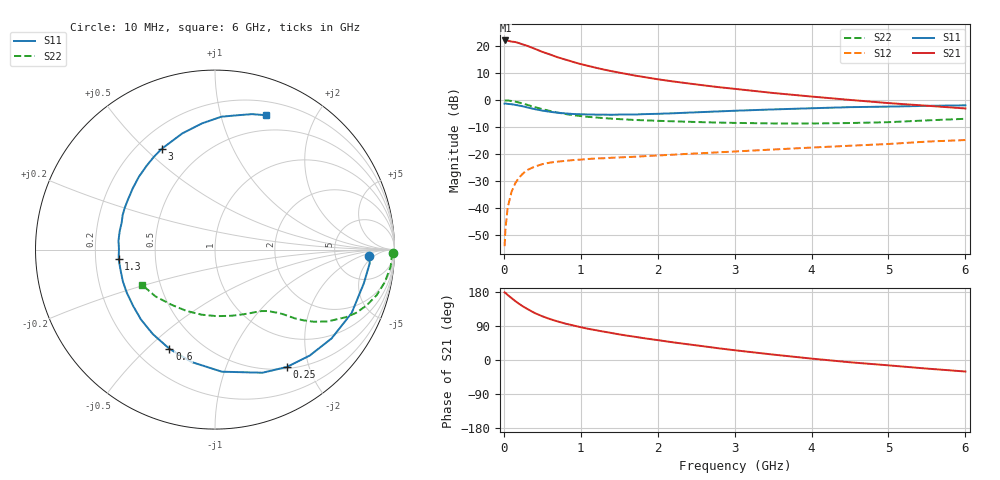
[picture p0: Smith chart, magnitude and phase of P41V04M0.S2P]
! SIEMENS Small Signal Semiconductors
! BFP182
! Si NPN RF Bipolar Junction Transistor in SOT143
! VCE = 1 V  IC = 4 mA
! Common Emitter S-Parameters:  March  1996
# GHz  S  MA  R  50
!  f  S11  S21  S12  S22
! GHz  MAG  ANG  MAG  ANG  MAG  ANG  MAG  ANG
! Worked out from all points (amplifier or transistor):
!   36 points, 10 MHz to 6 GHz, reference 50 ohm
!   highest |S21| = 22.0 dB at 20 MHz (marker M1)
!   |S21| within 3 dB of that: start of sweep to 395.9 MHz
!   unconditionally stable (mu >= 1): 1.622 GHz to end of sweep
!   at 250 MHz: K = 0.20, MSG = 23.8 dB, |S12| = -27.1 dB
!   at 1.4 GHz: K = 0.90, MSG = 16.0 dB, |S12| = -21.3 dB
!   at 6 GHz: K = 1.02, MAG = 4.9 dB, |S12| = -14.8 dB
!   S11 on the Smith chart (normalised r, x): 10 MHz: 12, -3; 250 MHz: 0.52, -1.66; 600 MHz: 0.34, -0.59; 1.3 GHz: 0.30, -0.04; 3 GHz: 0.30, +0.56; 6 GHz: 0.33, +1.40
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0.01  0.8606 -2.4  12.42 178.6  0.002 81.2  0.9895 -1.1
0.02  0.8652 -5.1  12.65 177.2  0.004 88.8  0.9859 -2.2
0.05  0.8504 -12.7  12.52 171.6  0.0104 84.8  0.9835 -5.5
0.15  0.8166 -37.3  11.81 155.3  0.0293 69.9  0.9356 -15.8
0.2  0.7919 -48.2  11.27 148.0  0.0374 65.0  0.9003 -20.2
0.25  0.7669 -58.5  10.62 141.2  0.0442 59.3  0.8621 -24.1
0.3  0.7353 -68.9  10.12 135.3  0.0506 55.2  0.8211 -27.3
0.4  0.6813 -86.8  8.91 124.1  0.059 48.1  0.7446 -32.5
0.5  0.6397 -101.8  7.788 115.4  0.0655 42.0  0.6805 -36.2
0.6  0.6082 -114.7  6.969 108.0  0.07 38.2  0.6298 -38.7
0.7  0.5844 -126.4  6.183 101.7  0.073 35.2  0.5877 -40.7
0.8  0.5674 -136.6  5.608 96.0  0.0753 32.6  0.5539 -42.1
1  0.5472 -153.9  4.626 86.5  0.0795 29.6  0.5069 -44.5
1.1  0.543 -161.1  4.276 82.2  0.0818 28.6  0.4904 -45.7
1.3  0.5392 -174.4  3.665 74.8  0.0844 26.7  0.4647 -48.0
1.7  0.5409 164.1  2.848 61.4  0.0898 25.7  0.4294 -52.9
2.2  0.5709 143.6  2.212 46.6  0.098 25.2  0.4058 -60.6
3  0.6356 117.7  1.615 25.8  0.1123 24.1  0.3791 -76.6
3.5  0.6726 105.7  1.354 14.3  0.1223 22.6  0.3709 -88.5
4.5  0.7411 87.3  1.008 -6.0  0.1436 18.7  0.377 -115.2
5.5  0.7826 74.7  0.787 -22.7  0.1711 14.0  0.4218 -141.8
6  0.8011 69.1  0.701 -30.4  0.1829 10.0  0.4514 -154.2
